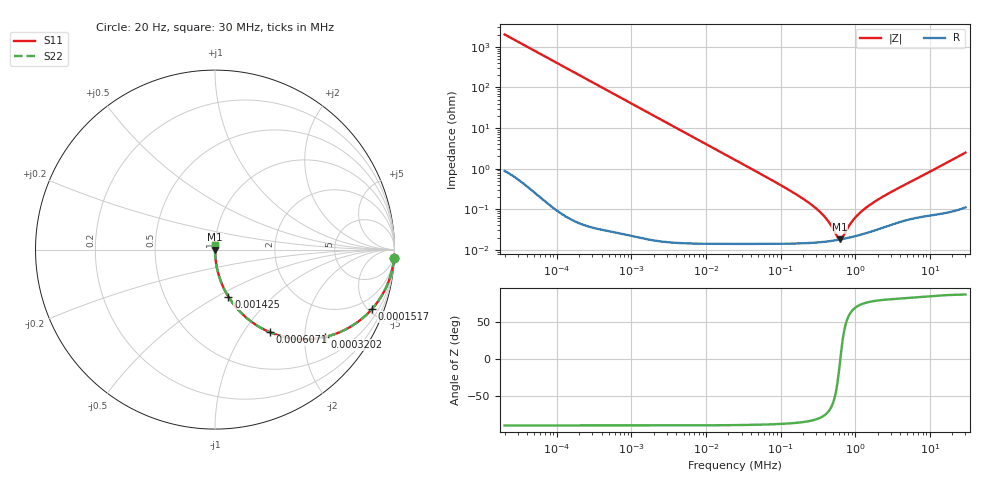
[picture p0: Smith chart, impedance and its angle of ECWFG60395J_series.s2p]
!  *** S-Parameter ***
!  Copyright (C) Panasonic Industry
!  Plastic Film Capacitor (ECWFG)
!  Parts No. ECWFG60395J
!  Connection Mode : Series
!  1  o---||---o  2
!  GND o--------o GND
!  Conditions : Temperature = 20   DC Bias = 0 V
! Frequency Range : 20 Hz  -  30 MHz  [ 401 Steps ]
# Hz S RI R 50
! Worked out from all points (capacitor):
!   401 points, 20 Hz to 30 MHz, reference 50 ohm
!   read as one part in series: C = 3.95 uF near 21.47 Hz
!   lowest |Z| = 18 mohm at 622.5 kHz (marker M1)
!   series resonance near 631.7 kHz, so ESL is about 16 nH
!   S11 on the Smith chart (normalised r, x): 20 Hz: 1, -40; 151.7 Hz: 1.00, -5.31; 320.2 Hz: 1.00, -2.52; 607.1 Hz: 1.00, -1.33; 1.425 kHz: 1.00, -0.57; 30 MHz: 1.00, +0.05
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20  0.9975 -0.0495  0.00248 0.0495  0.00248 0.0495  0.9975 -0.0495
60.21117  0.9781 -0.1461  0.0219 0.1461  0.0219 0.1461  0.9781 -0.1461
151.748  0.8759 -0.3296  0.1241 0.3296  0.1241 0.3296  0.8759 -0.3296
216.5336  0.7761 -0.4167  0.2239 0.4167  0.2239 0.4167  0.7761 -0.4167
320.1605  0.6133 -0.4869  0.3867 0.4869  0.3867 0.4869  0.6133 -0.4869
607.1443  0.3062 -0.4607  0.6938 0.4607  0.6938 0.4607  0.3062 -0.4607
930.1964  0.1584 -0.3648  0.8416 0.3648  0.8416 0.3648  0.1584 -0.3648
1425.139  0.0743 -0.2619  0.9257 0.2619  0.9257 0.2619  0.0743 -0.2619
2344.34  0.0289 -0.1671  0.9711 0.1671  0.9711 0.1671  0.0289 -0.1671
6122.189  0.00446 -0.0656  0.9955 0.0656  0.9955 0.0656  0.00446 -0.0656
24494.9  0.00041 -0.0164  0.9996 0.0164  0.9996 0.0164  0.00041 -0.0164
125697.3  0.000151 -0.00308  0.9998 0.00308  0.9998 0.00308  0.000151 -0.00308
265198.4  0.00015 -0.00125  0.9998 0.00125  0.9998 0.00125  0.00015 -0.00125
406306.4  0.00016 -0.000575  0.9998 0.000575  0.9998 0.000575  0.00016 -0.000575
579770.3  0.000175 -0.000107  0.9998 0.000107  0.9998 0.000107  0.000175 -0.000107
622495.7  0.000179 -1.82e-05  0.9998 1.82e-05  0.9998 1.82e-05  0.000179 -1.82e-05
668369.8  0.000184 7.04e-05  0.9998 -7.04e-05  0.9998 -7.04e-05  0.000184 7.04e-05
888257.1  0.000206 0.000428  0.9998 -0.000428  0.9998 -0.000428  0.000206 0.000428
1180485  0.000236 0.00081  0.9998 -0.00081  0.9998 -0.00081  0.000236 0.00081
1684468  0.000287 0.00136  0.9997 -0.00136  0.9997 -0.00136  0.000287 0.00136
2871218  0.000404 0.00248  0.9996 -0.00248  0.9996 -0.00248  0.000404 0.00248
3e7  0.00172 0.0247  0.9983 -0.0247  0.9983 -0.0247  0.00172 0.0247
